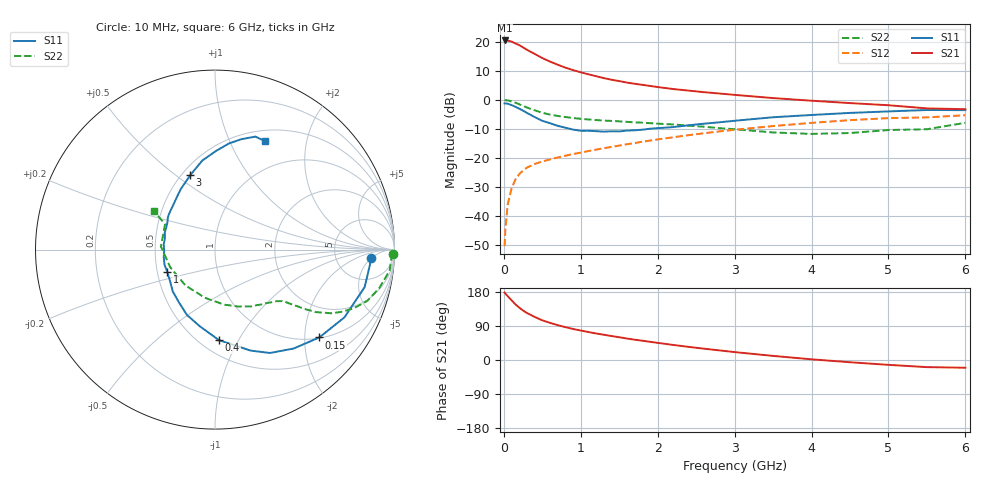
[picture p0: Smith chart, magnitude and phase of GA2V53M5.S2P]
! Infineon Technologies  Discrete & RF Semiconductors
! BF775
! Si NPN RF Bipolar Junction Transistor in SOT23
! VCE = 2.5 V  IC = 3.5 mA
! Common Emitter S-Parameters:  May  1996
# GHz  S  MA  R  50
!  f  S11  S21  S12  S22
! GHz  MAG  ANG  MAG  ANG  MAG  ANG  MAG  ANG
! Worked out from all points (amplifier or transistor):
!   36 points, 10 MHz to 6 GHz, reference 50 ohm
!   highest |S21| = 20.5 dB at 10 MHz (marker M1)
!   |S21| within 3 dB of that: start of sweep to 286.4 MHz
!   unconditionally stable (mu >= 1): 903.3 MHz to 3.845 GHz; 5.435 GHz to 5.664 GHz
!   at 250 MHz: K = 0.40, MSG = 21.2 dB, |S12| = -24.4 dB
!   at 1.4 GHz: K = 1.14, MAG = 9.3 dB, |S12| = -16.2 dB
!   at 6 GHz: K = 0.99, MSG = 1.0 dB, |S12| = -5.3 dB
!   S11 on the Smith chart (normalised r, x): 10 MHz: 13, -5; 150 MHz: 1.02, -2.36; 400 MHz: 0.62, -0.83; 1 GHz: 0.57, -0.15; 3 GHz: 0.55, +0.56; 6 GHz: 0.63, +1.37
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0.01  0.8692 -3.0  10.58 177.9  0.003 88.4  0.9937 -1.4
0.02  0.8672 -5.7  10.42 175.2  0.0059 85.1  0.9847 -2.7
0.05  0.8596 -14.1  10.51 168.5  0.0157 81.2  0.9799 -6.9
0.1  0.8143 -27.6  10.13 157.7  0.0296 75.5  0.94 -13.2
0.15  0.7598 -40.1  9.394 147.0  0.0423 69.0  0.8954 -18.6
0.2  0.7042 -51.5  8.797 138.3  0.0523 63.7  0.8397 -22.9
0.25  0.6524 -62.0  8.023 130.5  0.0605 59.6  0.7841 -26.3
0.3  0.5965 -70.6  7.303 124.1  0.0678 57.0  0.7386 -28.7
0.4  0.5054 -87.4  6.207 113.7  0.0783 53.3  0.6608 -31.8
0.5  0.4352 -101.3  5.261 104.7  0.0866 51.3  0.5984 -33.5
0.6  0.3963 -113.2  4.574 98.0  0.0941 50.6  0.5577 -34.5
0.8  0.3314 -135.2  3.597 86.7  0.1088 50.4  0.5057 -36.1
1  0.2934 -154.9  2.988 77.7  0.1231 51.3  0.4715 -37.5
1.1  0.2937 -163.4  2.759 73.8  0.1311 51.6  0.4592 -38.7
1.3  0.2832 -178.9  2.374 66.6  0.147 51.8  0.4398 -41.0
1.6  0.2955 161.2  1.986 56.7  0.1717 51.6  0.4178 -45.4
2.2  0.3393 133.6  1.538 39.8  0.2263 49.4  0.3769 -57.0
3  0.4364 108.5  1.219 20.9  0.3052 42.8  0.3116 -80.3
3.5  0.5013 98.1  1.074 10.8  0.3534 37.3  0.2742 -101.8
4.5  0.5957 82.6  0.88 -5.9  0.447 24.5  0.2681 -158.3
5.5  0.6687 70.3  0.713 -18.8  0.499 9.4  0.3117 153.2
6  0.6652 65.1  0.69 -20.4  0.5436 5.3  0.4021 147.6
